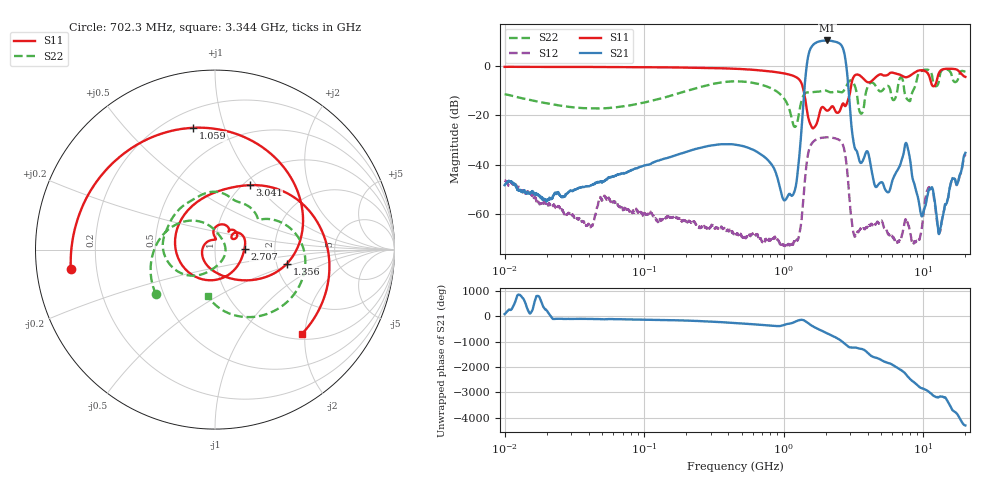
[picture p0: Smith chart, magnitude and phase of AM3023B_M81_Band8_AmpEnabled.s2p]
!Agilent Technologies,E8364B,MY43040894,A.07.50.67
!Agilent E8364B: A.07.50.67
!Date: Tuesday, October 27, 2020 10:44:41
!Correction: S11(Full 2 Port(1,2))
!S21(Full 2 Port(1,2))
!S12(Full 2 Port(1,2))
!S22(Full 2 Port(1,2))
!S2P File: Measurements: S11, S21, S12, S22:Log Frequency Sweep
# Hz S  dB  R 50
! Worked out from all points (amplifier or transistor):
!   3201 points, 10 MHz to 20 GHz, reference 50 ohm
!   highest |S21| = 10.4 dB at 2.055 GHz (marker M1)
!   |S21| within 3 dB of that: 1.564 GHz to 2.645 GHz (1.081 GHz wide, 51.4 % of centre)
!   unconditionally stable (mu >= 1): start of sweep to end of sweep
!   at 35.47 MHz: K = 15122.28, MAG = -38.1 dB, |S12| = -62.6 dB
!   at 447.2 MHz: K = 8179.42, MAG = -24.0 dB, |S12| = -68.0 dB
!   at 20 GHz: K = 456.90, MAG = -29.3 dB, |S12| = -35.7 dB
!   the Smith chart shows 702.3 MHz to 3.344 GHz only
!   S11 on the Smith chart (normalised r, x): 702.3 MHz: 0.10, -0.07; 1.059 GHz: 0.31, +0.79; 1.356 GHz: 2.28, -0.43; 2.707 GHz: 1.39, +0.02; 3.041 GHz: 1.07, +0.92; 3.344 GHz: 1.12, -1.93
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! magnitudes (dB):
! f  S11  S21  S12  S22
! 10 MHz  -0.3  -48.2  -46.3  -11.4
! 35.55 MHz  -0.4  -49.1  -62.8  -17.0
! 52.99 MHz  -0.4  -46.1  -53.4  -17.1
! 126.1 MHz  -0.5  -38.3  -63.1  -13.4
! 447.2 MHz  -1.1  -31.8  -68.0  -6.2
! 702.3 MHz  -1.8  -36.2  -71.3  -7.7
! 1.059 GHz  -3.2  -53.1  -72.3  -15.3
! 1.216 GHz  -4.4  -49.0  -71.1  -24.5
! 1.356 GHz  -7.8  -21.6  -58.8  -13.1
! 1.467 GHz  -18.1  1.1  -38.3  -10.7
! 1.59 GHz  -24.8  8.0  -31.3  -10.6
! 2.055 GHz  -18.1  10.4  -28.8  -10.1
! 2.707 GHz  -15.7  5.5  -33.7  -9.8
! 3.041 GHz  -7.8  -23.3  -61.1  -5.8
! 3.344 GHz  -3.4  -34.6  -67.5  -11.6
! 3.591 GHz  -4.3  -39.2  -65.6  -19.3
! 5.639 GHz  -3.3  -51.1  -68.4  -8.2
! 7.588 GHz  -4.5  -31.5  -62.3  -13.1
! 9.646 GHz  -1.7  -60.3  -67.4  -2.0
! 11.07 GHz  -4.5  -49.6  -49.1  -1.8
! 13.1 GHz  -2.2  -66.9  -67.2  -3.7
! 20 GHz  -4.4  -35.1  -35.7  -2.3
